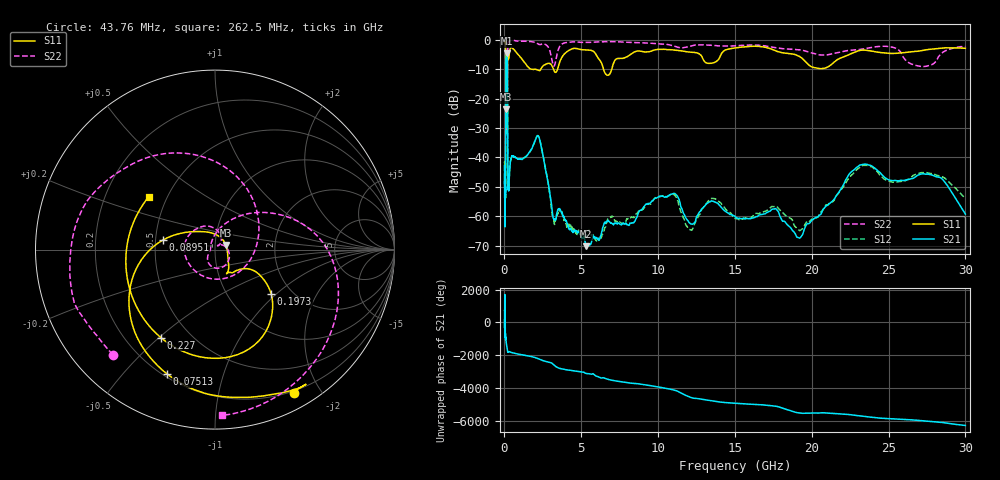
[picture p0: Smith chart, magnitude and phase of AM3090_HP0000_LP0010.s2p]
! Date/Time: Thu, Feb 28, 2019 1:52 PM
! Network Analyzer: Agilent Technologies E8364B Rev: A.07.50.67
! Sweep from 0.010 to 30.000 GHz, 1601 Points, Sweep Type: LOG
! Power Supply: 5.023 V, 0.002 A
# Hz S DB R 50
!freq MagS11 AngS11 MagS21 AngS21 MagS12 AngS12 MagS22 AngS22
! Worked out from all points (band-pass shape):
!   1601 points, 10 MHz to 30 GHz, reference 50 ohm
!   highest |S21| = -4.54 dB at 136.3 MHz (marker M1); lowest = -70.2 dB at 5.311 GHz (marker M2)
!   |S21| within 3 dB of the highest: 98.13 MHz to 183.7 MHz (85.59 MHz wide, 60.7 % of centre)
!   lowest |S11| = -23.6 dB at 97.46 MHz (marker M3), VSWR 1.14, Z = 56.4 + j2.94 ohm
!   |S11| at or under -10 dB: 2.043 GHz to 2.362 GHz (319.4 MHz wide, 14.5 % of centre); 3.196 GHz to 3.453 GHz (256.7 MHz wide, 7.72 % of centre); 6.454 GHz to 6.981 GHz (526.7 MHz wide, 7.84 % of centre)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
!   |S22| runs from -32.0 to -0.2 dB; largest |S21 - S12| = 0.014
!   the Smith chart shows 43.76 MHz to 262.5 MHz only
!   S11 on the Smith chart (normalised r, x): 43.76 MHz: 0.18, -1.67; 75.13 MHz: 0.22, -0.66; 89.51 MHz: 0.55, +0.06; 197.3 MHz: 1.57, -0.93; 227 MHz: 0.35, -0.51; 262.5 MHz: 0.40, +0.30
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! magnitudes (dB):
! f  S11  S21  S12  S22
! 10 MHz  -0.2  -42.8  -42.8  -0.6
! 38.04 MHz  -0.5  -59.5  -59.4  -1.4
! 43.76 MHz  -0.8  -57.7  -58.6  -1.8
! 75.13 MHz  -2.6  -44.6  -44.0  -4.9
! 89.51 MHz  -10.6  -14.8  -14.7  -15.5
! 97.46 MHz  -23.6  -7.8  -7.8  -15.5
! 136.3 MHz  -16.3  -4.5  -4.5  -25.7
! 144.7 MHz  -15.9  -4.6  -4.6  -21.1
! 177.7 MHz  -13.9  -6.4  -6.4  -31.8
! 197.3 MHz  -7.9  -15.0  -15.0  -11.3
! 227 MHz  -4.8  -50.4  -49.8  -1.7
! 262.5 MHz  -6.5  -50.8  -50.2  -0.7
! 550.5 MHz  -3.0  -39.5  -39.7  -0.3
! 2.084 GHz  -10.1  -33.1  -33.0  -1.0
! 3.204 GHz  -10.1  -60.9  -60.9  -8.9
! 5.311 GHz  -3.4  -70.2  -66.9  -0.8
! 7.926 GHz  -5.9  -62.4  -61.4  -0.8
! 10.81 GHz  -3.3  -52.6  -52.6  -1.7
! 12.07 GHz  -4.1  -62.4  -64.6  -2.2
! 19.22 GHz  -5.6  -67.5  -64.9  -3.4
! 23.48 GHz  -3.5  -42.3  -42.7  -2.9
! 30 GHz  -2.8  -59.2  -53.9  -2.2
